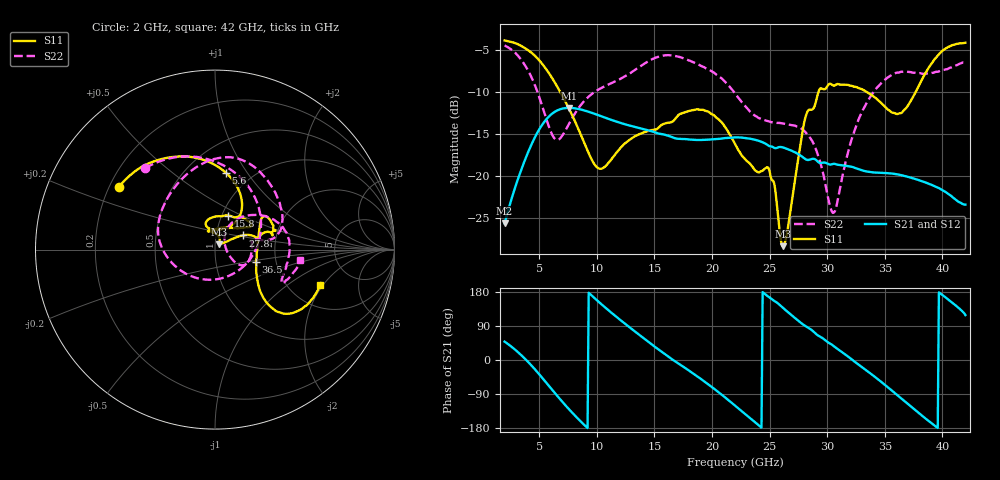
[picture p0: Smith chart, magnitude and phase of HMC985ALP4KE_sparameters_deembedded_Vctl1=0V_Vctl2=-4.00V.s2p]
!s2p File: Measurements: S11, S21, S12, S22
# GHz S dB R 50.0
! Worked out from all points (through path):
!   401 points, 2 GHz to 42 GHz, reference 50 ohm
!   highest |S21| = -11.91 dB at 7.6 GHz (marker M1); lowest = -25.7 dB at 2 GHz (marker M2)
!   lowest |S11| = -28.4 dB at 26.2 GHz (marker M3), VSWR 1.08, Z = 52.3 + j3.16 ohm
!   |S11| at or under -10 dB: 6.822 GHz to 29.25 GHz (22.43 GHz wide, 124 % of centre); 33.42 GHz to 37.69 GHz (4.272 GHz wide, 12 % of centre)
!   |S22| runs from -24.4 to -4.5 dB; largest |S21 - S12| = 0.00019
!   S11 on the Smith chart (normalised r, x): 2 GHz: 0.24, +0.28; 5.6 GHz: 0.76, +0.80; 15.8 GHz: 1.07, +0.42; 27.8 GHz: 1.34, +0.22; 36.5 GHz: 1.57, -0.23; 42 GHz: 2.95, -1.89
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2  -3.88 147.0  -25.67 48.5  -25.68 48.6  -4.47 130.5
3.6  -4.66 120.3  -18.71 8.3  -18.71 8.3  -6.49 85.0
4.6  -5.66 101.5  -15.49 -23.5  -15.49 -23.5  -9.11 47.8
5.6  -7.28 81.9  -13.30 -59.2  -13.31 -59.2  -13.13 -3.7
6.5  -9.21 66.5  -12.26 -92.2  -12.26 -92.2  -15.70 -69.4
7.6  -12.03 54.7  -11.91 -130.3  -11.91 -130.3  -13.78 -136.3
8.7  -15.38 55.0  -12.13 -164.9  -12.13 -164.9  -11.43 -170.6
10.4  -19.15 89.6  -12.91 147.2  -12.91 147.2  -9.53 162.1
15.4  -14.22 75.7  -14.97 27.1  -14.98 27.1  -5.80 86.5
15.8  -13.83 68.7  -15.07 18.2  -15.08 18.1  -5.67 81.5
19.3  -12.17 33.6  -15.71 -55.7  -15.72 -55.7  -7.04 35.8
22  -16.19 51.2  -15.42 -120.3  -15.43 -120.4  -10.18 10.2
24.9  -19.04 104.6  -16.40 167.0  -16.40 167.0  -13.50 13.2
26.2  -28.38 52.4  -16.63 136.6  -16.64 136.6  -13.78 -3.2
27.8  -15.23 27.2  -17.69 96.1  -17.69 96.1  -14.40 -25.3
28.7  -12.11 12.6  -17.98 78.0  -17.98 77.9  -15.85 -31.9
30.6  -9.26 19.6  -18.57 36.0  -18.57 36.0  -24.36 20.8
32.8  -9.59 33.9  -19.25 -13.9  -19.25 -13.9  -13.05 52.3
35.4  -12.22 11.7  -19.70 -75.2  -19.70 -75.2  -8.18 20.4
36.5  -12.47 -16.6  -19.94 -103.1  -19.94 -103.1  -7.60 6.5
39.5  -5.86 -43.7  -21.33 -176.9  -21.33 -177.0  -7.61 -26.1
42  -4.15 -18.6  -23.43 118.6  -23.44 118.5  -6.40 -6.8
